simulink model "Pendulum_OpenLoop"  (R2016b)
settings: Solver=ode1  StartTime=0.0  StopTime=20  FixedStep=0.001  RelTol=1e-3
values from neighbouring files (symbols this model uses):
  c = 0.5    [PendulumParameters.m]
  Dtheta_0 = 0    [PendulumParameters.m]
  g = 9.81    [PendulumParameters.m]
  L = 0.5    [PendulumParameters.m]
  m = 2    [PendulumParameters.m]
  theta_0 = 0    [PendulumParameters.m]
undefined symbols (not defined in the file or in its folder): sigbuilder_block

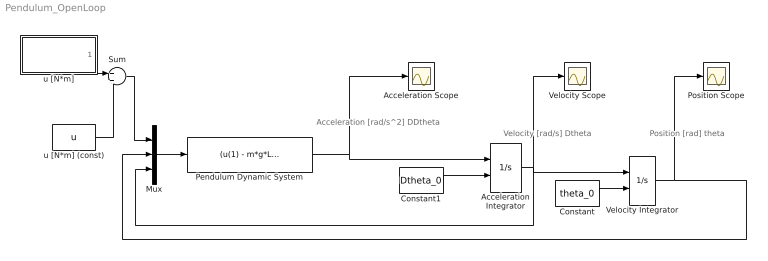
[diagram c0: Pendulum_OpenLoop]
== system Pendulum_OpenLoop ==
  note: Position [rad] theta
  note: Velocity [rad/s] Dtheta
  note: Acceleration [rad/s^2] DDtheta
  Acceleration Integrator : Integrator  InitialConditionSource=external
  "Acceleration Scope " : Scope
  Constant : Constant  Value=theta_0
  Constant1 : Constant  Value=Dtheta_0
  Mux : Mux  Inputs=3
  Pendulum Dynamic System : Fcn  Expr=(u(1) - m*g*L*sin(u(2)) - c*u(3)) / (m*L*L)
  Position Scope : Scope
  Sum : Sum  Inputs=+|+
  Velocity Integrator : Integrator  InitialConditionSource=external
  Velocity Scope : Scope
  u [N*m] : Subsystem  Tag=STV Subsys  LoadFcn=sigbuilder_block('load');  StartFcn=sigbuilder_block('start');  StopFcn=sigbuilder_block('stop');  ClipboardFcn=sigbuilder_block('clipboard');
  u [N*m] (const) : Constant  Value=u
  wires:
  Velocity Integrator/1 -> Position Scope/1, Mux/2
  Mux/1 -> Pendulum Dynamic System/1
  Acceleration Integrator/1 -> Mux/3, Velocity Scope/1, Velocity Integrator/1
  Constant/1 -> Velocity Integrator/2
  Constant1/1 -> Acceleration Integrator/2
  Pendulum Dynamic System/1 -> "Acceleration Scope "/1, Acceleration Integrator/1
  u [N*m]/1(Signal 1) -> Sum/1
  u [N*m] (const)/1 -> Sum/2
  Sum/1 -> Mux/1

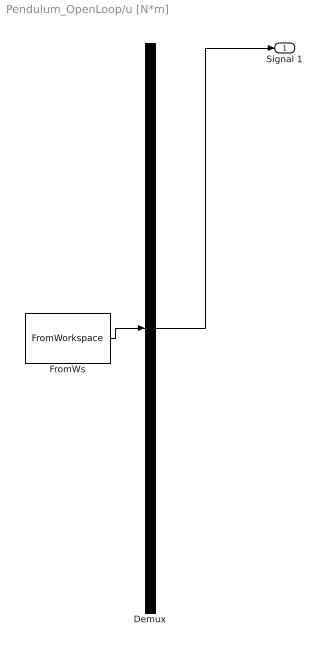
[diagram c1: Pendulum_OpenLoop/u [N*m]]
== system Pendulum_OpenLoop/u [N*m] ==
  Demux : Demux  Tag=STV Demux  Outputs=1
  FromWs : FromWorkspace  Tag=STV FromWs  VariableName=tuvar  SampleTime=0
  Signal 1 : Outport  Tag=STV Outport
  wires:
  Demux/1 -> Signal 1/1
  FromWs/1 -> Demux/1
